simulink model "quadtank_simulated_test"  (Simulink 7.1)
settings: Solver=ode45  StartTime=0.0  StopTime=150  FixedStep=0.01  RelTol=1e-6
PreLoadFcn:
  | init_quadtank
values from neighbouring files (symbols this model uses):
  W1 = eye(2)    [init_quadtank.m]
  W2 = eye(2)    [init_quadtank.m]
libraries: cstblocks x2, tank x1

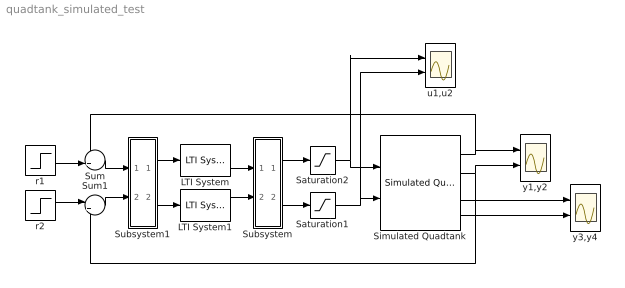
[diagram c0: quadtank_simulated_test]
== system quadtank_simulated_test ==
  LTI System : cstblocks/LTI System  SystemSampleTime=-1  sys=C1  IC=[]
  LTI System1 : cstblocks/LTI System  SystemSampleTime=-1  sys=C2  IC=[]
  Saturation1 : Saturate  UpperLimit=10  LowerLimit=0
  Saturation2 : Saturate  UpperLimit=10  LowerLimit=0
  Simulated Quadtank : tank/Simulated Quadtank  SystemSampleTime=-1  gamma1=0.7  gamma2=0.7
  Subsystem : Subsystem
  Subsystem1 : Subsystem
  Sum : Sum  Inputs=-+|
  Sum1 : Sum  Inputs=|+-
  r1 : Step  Time=50  Before=5  After=6  SampleTime=0
  r2 : Step  Time=100  Before=5  After=6  SampleTime=0
  u1,u2 : Scope  NumInputPorts=2
  y1,y2 : Scope  NumInputPorts=2
  y3,y4 : Scope  NumInputPorts=2
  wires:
  Simulated Quadtank/1 -> y1,y2/1, Sum/1
  Simulated Quadtank/2 -> y1,y2/2, Sum1/2
  r2/1 -> Sum1/1
  Simulated Quadtank/3 -> y3,y4/1
  Simulated Quadtank/4 -> y3,y4/2
  Saturation2/1 -> u1,u2/1, Simulated Quadtank/1
  Saturation1/1 -> u1,u2/2, Simulated Quadtank/2
  LTI System/1 -> Subsystem/1(In1)
  Subsystem1/1(Out1) -> LTI System/1
  Subsystem/1(Out1) -> Saturation2/1
  Subsystem/2(Out2) -> Saturation1/1
  Sum/1 -> Subsystem1/1(In1)
  Sum1/1 -> Subsystem1/2(In2)
  r1/1 -> Sum/2
  LTI System1/1 -> Subsystem/2(In2)
  Subsystem1/2(Out2) -> LTI System1/1

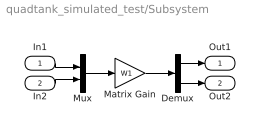
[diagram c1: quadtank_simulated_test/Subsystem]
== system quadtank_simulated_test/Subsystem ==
  In1 : Inport
  In2 : Inport  Port=2
  Demux : Demux  Outputs=2
  Matrix Gain : Gain  Gain=W1  Multiplication=Matrix(K*u)
  Mux : Mux  Inputs=2
  Out1 : Outport
  Out2 : Outport  Port=2
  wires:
  Demux/1 -> Out1/1
  In1/1 -> Mux/1
  Demux/2 -> Out2/1
  In2/1 -> Mux/2
  Mux/1 -> Matrix Gain/1
  Matrix Gain/1 -> Demux/1

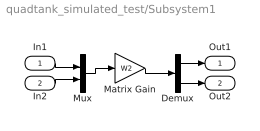
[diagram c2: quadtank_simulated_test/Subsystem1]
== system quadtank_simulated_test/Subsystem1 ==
  In1 : Inport
  In2 : Inport  Port=2
  Demux : Demux  Outputs=2
  Matrix Gain : Gain  Gain=W2  Multiplication=Matrix(K*u)
  Mux : Mux  Inputs=2
  Out1 : Outport
  Out2 : Outport  Port=2
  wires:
  Matrix Gain/1 -> Demux/1
  Mux/1 -> Matrix Gain/1
  In2/1 -> Mux/2
  Demux/2 -> Out2/1
  In1/1 -> Mux/1
  Demux/1 -> Out1/1
